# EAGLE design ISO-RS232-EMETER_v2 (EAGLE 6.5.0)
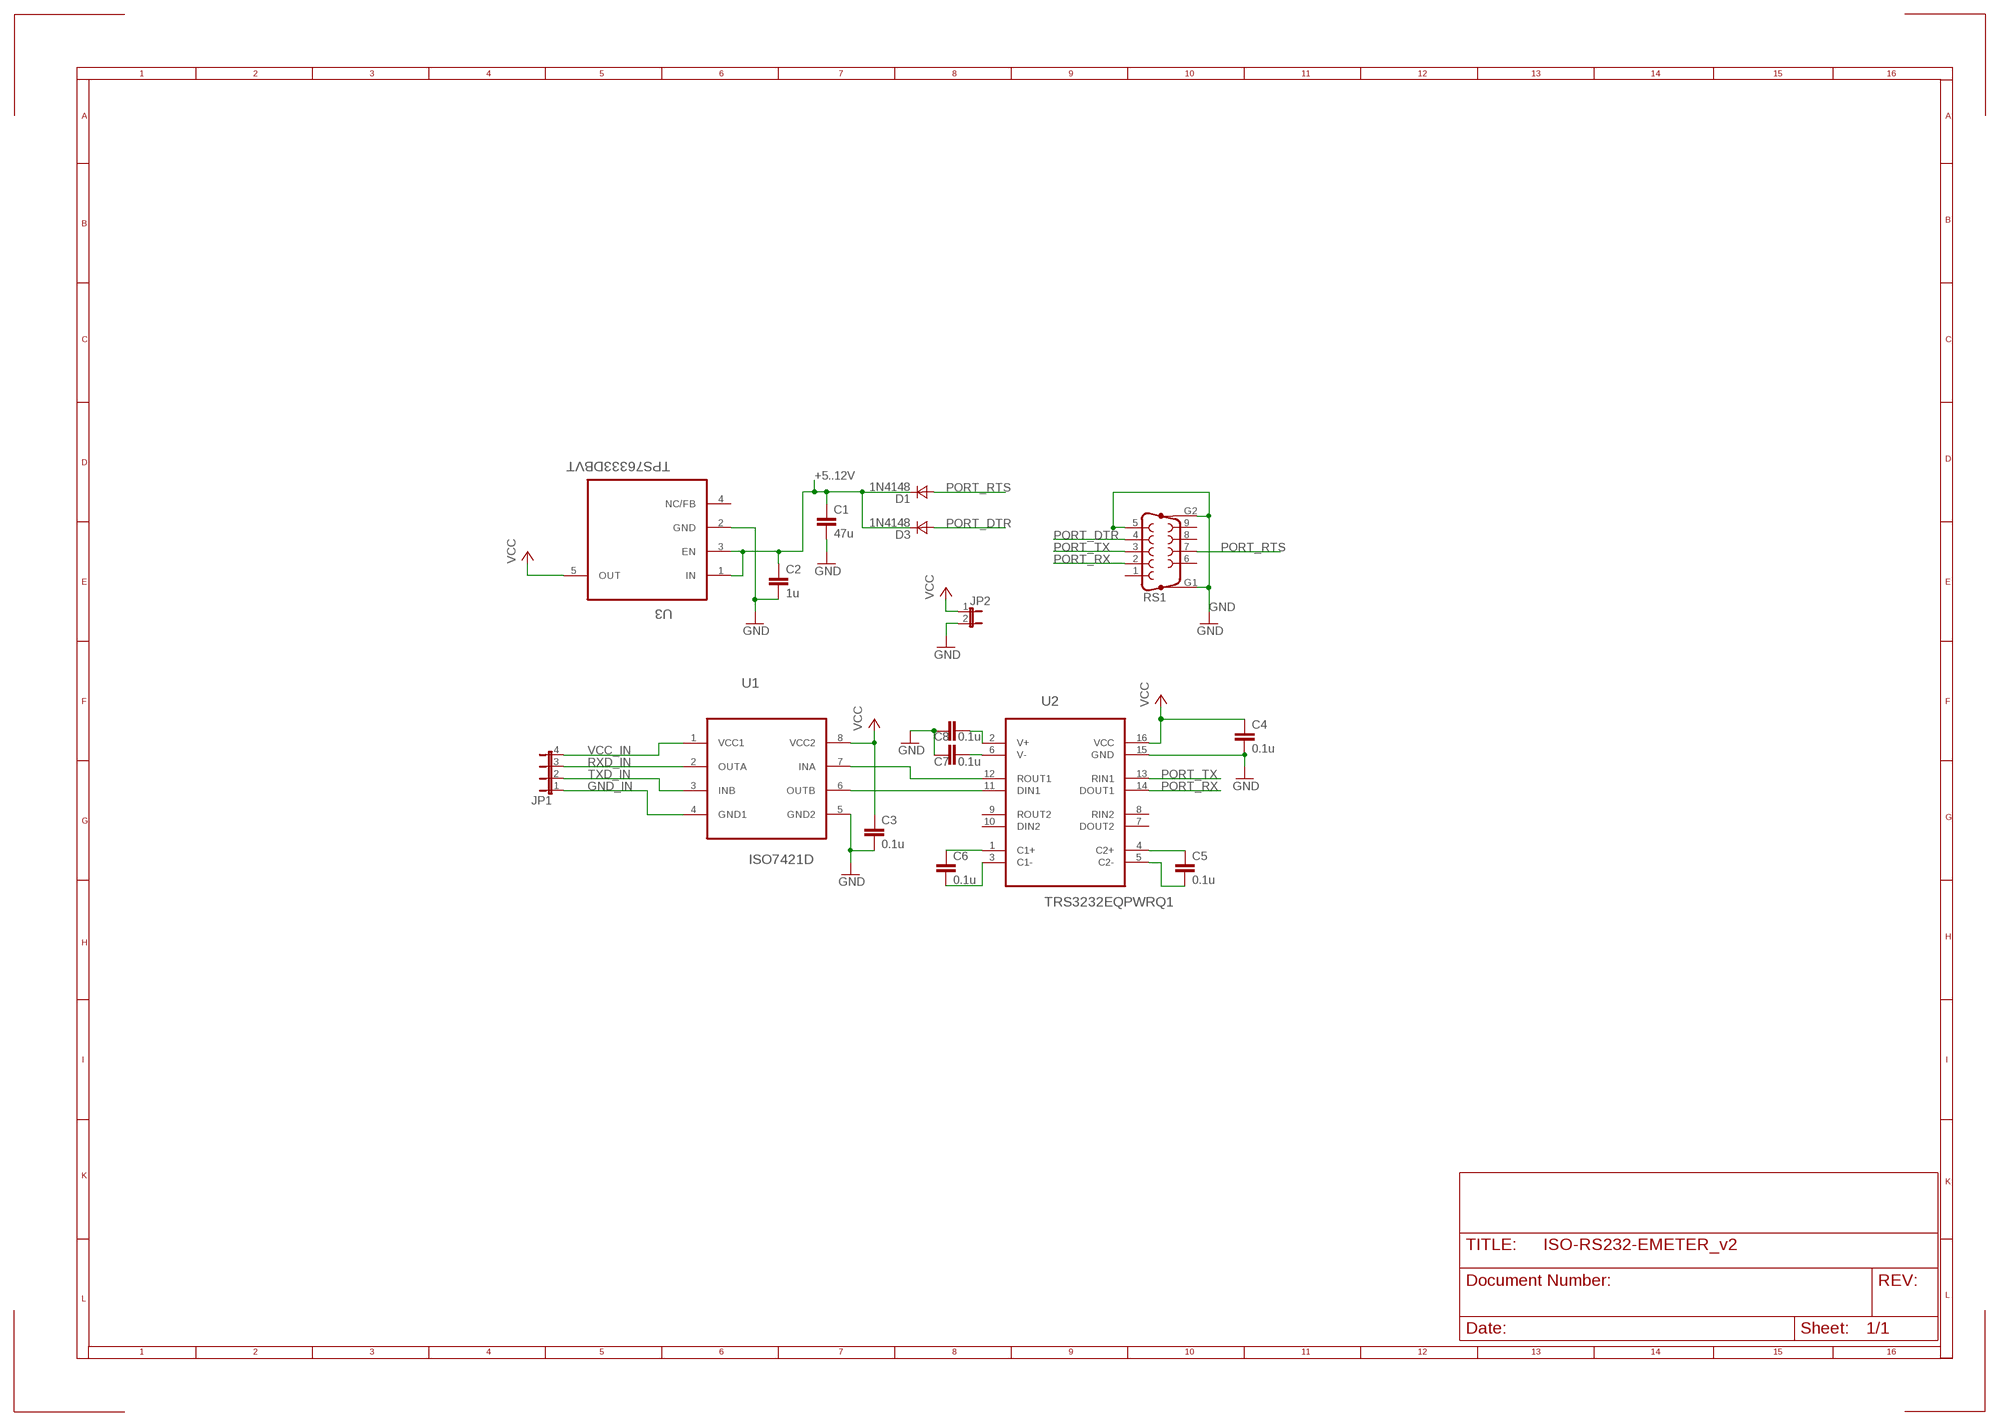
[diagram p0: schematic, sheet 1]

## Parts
C1  47u  C-EUC1206K  [C1206K]
C2  1u  C-EUC0603  [C0603]
C3  0.1u  C-EUC0603  [C0603]
C4  0.1u  C-EUC0603  [C0603]
C5  0.1u  C-EUC0603  [C0603]
C6  0.1u  C-EUC0603  [C0603]
C7  0.1u  C-EUC0603  [C0603]
C8  0.1u  C-EUC0603  [C0603]
D1  1N4148  DSOD323  [SOD323]
D3  1N4148  DSOD323  [SOD323]
JP1  JP4E  [JP4]
JP2  JP1E  [JP1]
RS1  F09VP  [F09VP]
U1  ISO7421D  [SOIC127P600X175-8N]
U2  TRS3232EQPWRQ1  [SOP65P640X120-16N]
U3  TPS76333DBVT  [SOT95P280X145-5N]

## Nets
+5..12V: C1.1 C2.1 D1.1(C) D3.1(C) U3.1(IN) U3.3(EN)
GND: C1.2 C2.2 C3.2 C4.2 C7.1 C8.1 JP2.2 RS1.5 RS1.G1 RS1.G2 U1.5(GND2) U2.15(GND) U3.2(GND)
GND_IN: JP1.1 U1.4(GND1)
N$4: C5.1 U2.4(C2+)
N$5: C5.2 U2.5(C2-)
N$6: C6.1 U2.1(C1+)
N$7: C6.2 U2.3(C1-)
N$8: U1.7(INA) U2.12(ROUT1)
N$9: U1.6(OUTB) U2.11(DIN1)
N$10: C8.2 U2.2(V+)
N$11: C7.2 U2.6(V-)
PORT_DTR: D3.2(A) RS1.4
PORT_RTS: D1.2(A) RS1.7
PORT_RX: RS1.2 U2.14(DOUT1)
PORT_TX: RS1.3 U2.13(RIN1)
RXD_IN: JP1.3 U1.2(OUTA)
TXD_IN: JP1.2 U1.3(INB)
VCC: C3.1 C4.1 JP2.1 U1.8(VCC2) U2.16(VCC) U3.5(OUT)
VCC_IN: JP1.4 U1.1(VCC1)
Unconnected: RS1.1 RS1.6 RS1.8 RS1.9 U2.7(DOUT2) U2.8(RIN2) U2.9(ROUT2) U2.10(DIN2) U3.4(NC/FB)

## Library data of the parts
C1 = rcl:C-EU: CAPACITOR, European symbol; DIGIKEY: 445-8047-1-ND
C2-C8 = rcl:C-EU: CAPACITOR, European symbol; DIGIKEY: 445-5956-1-ND
D1 D3 = zetex:D: DIODE; DIGIKEY: 1N4148WSFSCT-ND; MPN: CDSOD323-T05C; OC_FARNELL: 1824860; OC_NEWARK: 79R6078
JP1 = jumper:JP4E: JUMPER; DIGIKEY: 609-3319-ND
JP2 = jumper:JP1E: JUMPER; DIGIKEY: 609-4434-ND
RS1 = con-subd:F09VP: SUB-D; DIGIKEY: A32119-ND; OC_FARNELL: unknown; OC_NEWARK: unknown
U1 = Texas Instruments_By_element14_Batch_1:ISO7421D: Low-Power Dual Digital Isolators; DIGIKEY: 296-25187-5-ND; MPN: ISO7421D; OC_FARNELL: -; OC_NEWARK: 33R2484; PACKAGE: SOIC-8; SUPPLIER: Texas Instruments
U2 = Texas Instruments_By_element14_Batch_1:TRS3232EQPWRQ1: RS-232 LINE DRIVER/RECEIVER; DIGIKEY: 296-24863-1-ND; MPN: TRS3232EQPWRQ1; OC_FARNELL: -; OC_NEWARK: 09R6724; PACKAGE: TSSOP-16; SUPPLIER: Texas Instruments
U3 = Texas Instruments_By_element14_Batch_1:TPS76333DBVT: Low Power 150mA Low Dropout Linear Regulator; DIGIKEY: 296-11021-1-ND; MPN: TPS76333DBVT; OC_FARNELL: 8461376; OC_NEWARK: 96C8605; PACKAGE: SOT-23-5; SUPPLIER: Texas Instruments

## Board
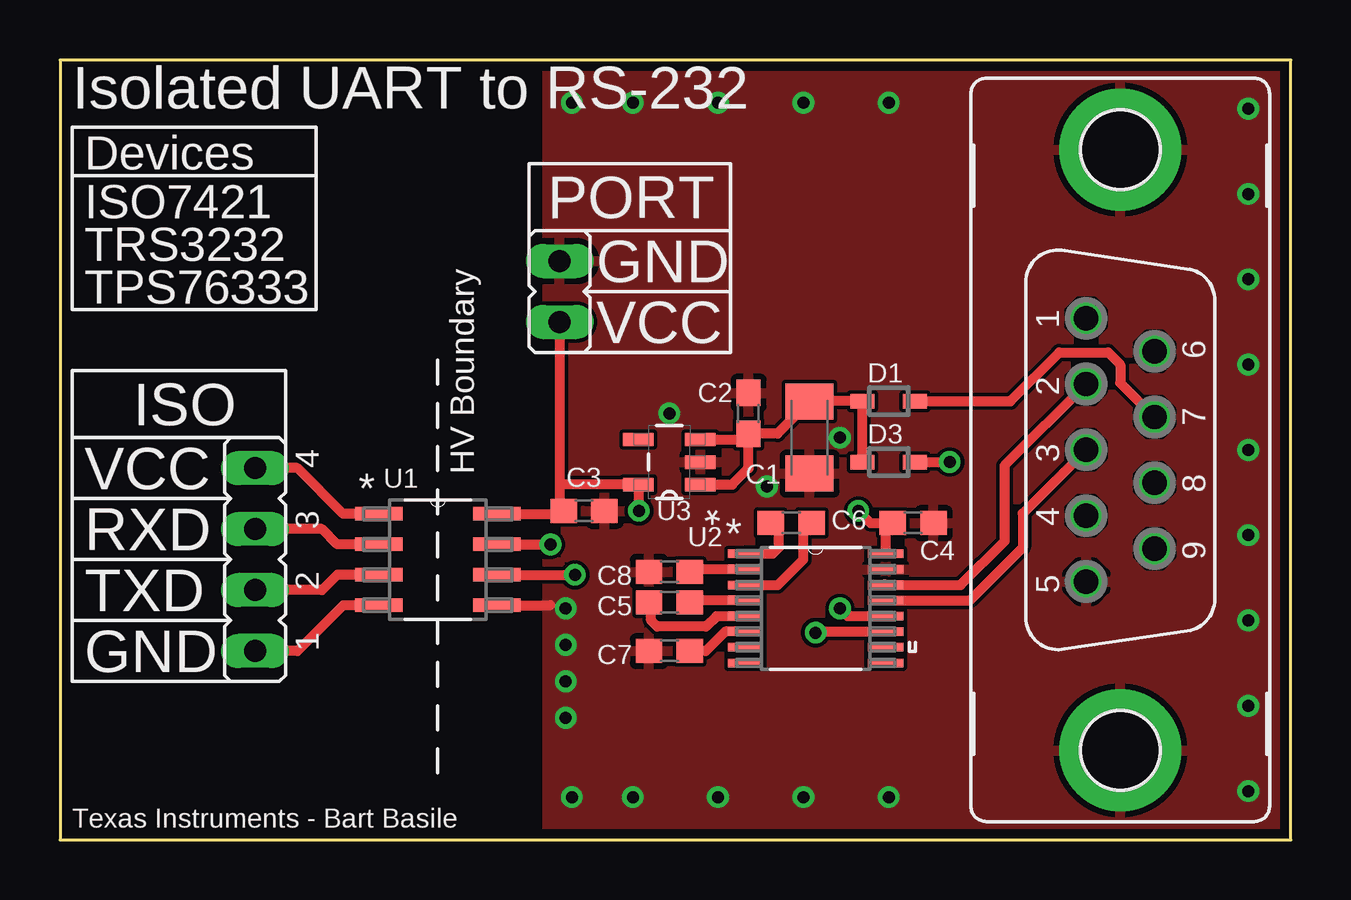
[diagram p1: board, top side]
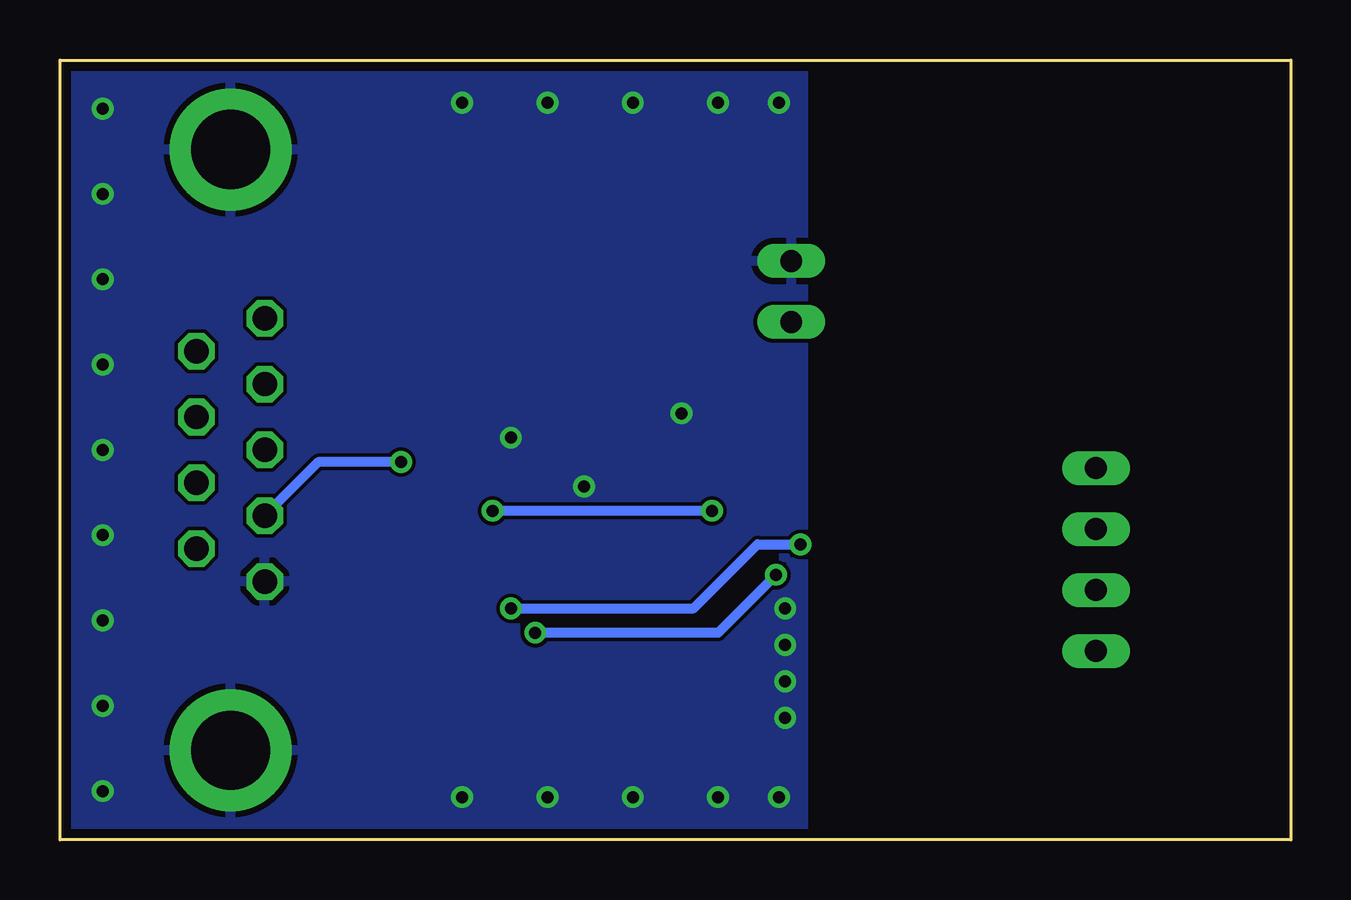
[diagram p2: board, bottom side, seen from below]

Size 51.31 x 32.51 mm. Coordinates in mm from the lower left corner, seen from the top.
Outline: 0,0 51.31,0 51.31,32.51 0,32.51 0,0
Copper layers (1*16): Top 0.035559375mm / dielectric 1.501140625mm / Bottom 0.035559375mm
Design rules "typical_4pcb *": minimum track width 10mil, minimum drill 15mil, track to track 6mil, track to pad 6mil, pad to pad 6mil, via to via 6mil, smd to smd 6mil, copper to edge 15mil, drill to drill 8mil, minimum pad ring 10mil, minimum via ring 8mil, stop-mask expansion 4mil, vias tented up to drill 20mil, thermal gap 10mil
bRestrict: 1 lines

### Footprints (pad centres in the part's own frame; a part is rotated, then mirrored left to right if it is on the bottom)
C1206K = smd 1.5 x 2: 1 -1.5,0; 2 1.5,0
C0603 = smd 1.1 x 1: 1 -0.85,0; 2 0.85,0
SOD323 = smd 1 x 0.6: 1 -1.1,0; 2 1.1,0
JP4 = drill 0.914 long: 1 -3.81,0; 2 -1.27,0; 3 1.27,0; 4 3.81,0
JP1 = drill 0.914 long: 1 0,-1.27; 2 0,1.27
F09VP = drill 1.016 octagon: 1 5.486,1.422; 2 2.743,1.422; 3 0,1.422; 4 -2.743,1.422; 5 -5.486,1.422; 6 4.115,-1.422; 7 1.372,-1.422; 8 -1.372,-1.422; 9 -4.115,-1.422 | drill 3.302 pad 5.08: G1 -12.522,0; G2 12.522,0
SOIC127P600X175-8N = smd 1.981 x 0.559: 1 -2.464,1.905; 2 -2.464,0.635; 3 -2.464,-0.635; 4 -2.464,-1.905; 5 2.464,-1.905; 6 2.464,-0.635; 7 2.464,0.635; 8 2.464,1.905
SOP65P640X120-16N = smd 1.473 x 0.356: 1 -2.921,2.286; 2 -2.921,1.626; 3 -2.921,0.965; 4 -2.921,0.33; 5 -2.921,-0.33; 6 -2.921,-0.965; 7 -2.921,-1.626; 8 -2.921,-2.286; 9 2.921,-2.286; 10 2.921,-1.626; 11 2.921,-0.965; 12 2.921,-0.33; 13 2.921,0.33; 14 2.921,0.965; 15 2.921,1.626; 16 2.921,2.286
SOT95P280X145-5N = smd 1.27 x 0.559: 1 -1.295,0.94; 2 -1.295,0; 3 -1.295,-0.94; 4 1.295,-0.94; 5 1.295,0.94

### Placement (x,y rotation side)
C1  31.24,16.76 270 top
C2  28.7,17.78 90 top
C3  21.84,13.72 0 top
C4  35.56,13.21 0 top
C5  25.4,9.91 180 top
C6  30.48,13.21 0 top
C7  25.4,7.87 0 top
C8  25.4,11.18 0 top
D1  34.54,18.29 0 top
D3  34.54,15.75 0 top
JP1  8.13,11.68 90 top
JP2  20.83,22.86 0 top
RS1  44.2,16.26 90 top
U1  15.75,11.68 0 top
U2  31.5,9.65 0 top
U3  25.4,15.75 180 top

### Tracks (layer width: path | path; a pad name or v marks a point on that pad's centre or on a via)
+5..12V
  Top 0.406: D3.1 D1.1 31.27,18.29 C1.1 29.91,16.93 C2.1 | U3.1 28.02,14.81 28.7,15.49 C2.1 | U3.3 28.46,16.69 C2.1
GND  (via drill 0.5)
  Top 0.406: U1.5 20.45,9.78
  other vias: 21.08,9.65 34.54,30.73 30.99,30.73 27.43,30.73 23.88,30.73 21.34,30.73 49.53,30.48 49.53,26.92 49.53,23.37 49.53,19.81 49.53,16.26 49.53,12.7 49.53,9.14 49.53,5.59 49.53,2.03 21.08,8.13 21.08,6.6 21.08,5.08 34.54,1.78 30.99,1.78 27.43,1.78 23.88,1.78 21.34,1.78 25.4,17.78 32.51,16.76 29.46,14.73
  pour Top: 20.32,32 50.8,32 50.8,0.51 20.32,0.51
  pour Bottom: 20.32,32 50.8,32 50.8,0.51 20.32,0.51
GND_IN
  Top 0.406: U1.4 11.81,9.78 9.91,7.87 JP1.1
N$4
  Top 0.406: U2.4 26.33,9.98 C5.1
N$5
  Top 0.406: U2.5 27.36,9.32 26.92,8.89 24.89,8.89 24.64,9.14 24.64,9.82 C5.2
N$6
  Top 0.406: U2.1 29.72,11.94 29.97,12.19 29.97,12.87 C6.1
N$7
  Top 0.406: U2.3 29.92,10.62 30.99,11.68 30.99,12.87 C6.2
N$8  (via drill 0.5)
  Top 0.406: U2.12 32.84,9.32 v32.51,9.65 | U1.7 v20.45,12.32
  Bottom 0.406: v32.51,9.65 24.89,9.65 22.23,12.32 v20.45,12.32
N$9  (via drill 0.5)
  Top 0.305: 34.47,8.64 U2.11
  Top 0.406: U1.6 v21.46,11.05 | v31.5,8.64 31.55,8.69 U2.11
  Bottom 0.406: v21.46,11.05 23.88,8.64 v31.5,8.64
N$10
  Top 0.406: U2.2 26.35,11.28 C8.2
N$11
  Top 0.406: U2.6 27.74,8.69 26.92,7.87 C7.2
PORT_DTR  (via drill 0.5)
  Top 0.406: D3.2 v37.08,15.75
  Bottom 0.406: v37.08,15.75 40.54,15.75 RS1.4
PORT_RTS
  Top 0.406: D1.2 39.62,18.29 41.66,20.32 43.69,20.32 44.2,19.81 44.2,19.05 RS1.7
PORT_RX
  Top 0.406: 34.37,10.67 U2.14 37.54,10.62 39.37,12.45 39.37,15.6 RS1.2
PORT_TX
  Top 0.406: U2.13 37.92,9.98 40.13,12.19 40.13,13.61 RS1.3
RXD_IN
  Top 0.406: U1.2 11.56,12.32 10.92,12.95 JP1.3
TXD_IN
  Top 0.406: U1.3 11.56,11.05 10.92,10.41 JP1.2
VCC  (via drill 0.5)
  Top 0.406: 34.54,13.37 C4.1 | U2.16 34.42,12.91 C4.1 | U1.8 20.87,13.59 arc90 C3.1 20.83,13.88 20.83,14.73 | v24.13,13.72 24.13,14.78 arc90 U3.5 20.9,14.81 20.83,14.73 | JP2.1 20.83,14.73 | v33.27,13.72 33.78,13.21 C4.1
  Bottom 0.406: v24.13,13.72 v33.27,13.72
VCC_IN
  Top 0.406: U1.1 11.81,13.59 9.91,15.49 JP1.4

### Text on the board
tPlace: Isolated UART to RS-232 | Devices | ISO7421 | PORT | TRS3232 | GND | TPS76333 | VCC | ISO | VCC | HV Boundary | RXD | TXD | GND | Texas Instruments - Bart Basile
